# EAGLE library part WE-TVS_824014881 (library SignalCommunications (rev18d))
WE-TVS TVS Diode – Super Speed Series Characteristics Operating temperature: –55 ºC to +85 °C for 824 014 x –40 ºC to +85 °C for 824 016 46 Low clamping voltage Very low capacitance Rail to Rail protection Epoxy flame resistant UL94-V0 RoHS, REACH and free of halogens Applications Super Speed data lines HDMI 1.3/1.4 DVI DisplayPort USB 3.0 SuperSpeed SATA GBit LAN Details see: http://katalog.we-online.de/en/pbs/WE-TVS-SS Created by Yingchun,Shan 2017-12-07 2017 (C) Wurth Elektronik
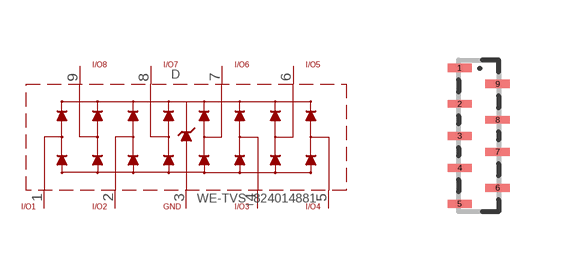
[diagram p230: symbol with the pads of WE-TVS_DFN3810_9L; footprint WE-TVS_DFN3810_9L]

Designator prefix D

## WE-TVS_824014881  [WE-TVS_DFN3810_9L]
1  1
2  2
3  GND
4  4
5  5
6  6
7  7
8  8
9  9

## Footprint WE-TVS_DFN3810_9L (pad centres in mm)
smd 0.6 x 0.2: 1 -0.475,1.7; 2 -0.475,0.8; 3 -0.475,0; 4 -0.475,-0.8; 5 -0.475,-1.7; 6 0.475,-1.3; 7 0.475,-0.4; 8 0.475,0.4; 9 0.475,1.3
